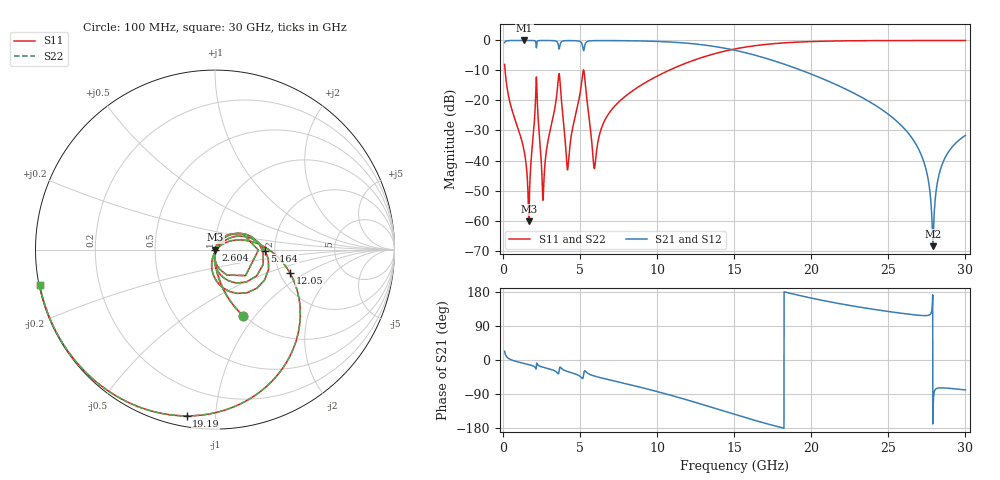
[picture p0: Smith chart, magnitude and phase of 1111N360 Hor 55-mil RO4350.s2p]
# GHz S MA R 50
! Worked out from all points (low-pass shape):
!   3201 points, 100 MHz to 30 GHz, reference 50 ohm
!   highest |S21| = -0.01 dB at 1.371 GHz (marker M1); lowest = -68.5 dB at 27.89 GHz (marker M2)
!   |S21| within 3 dB of the highest: start of sweep to 5.199 GHz; 5.253 GHz to 14.8 GHz (9.544 GHz wide, 95.2 % of centre)
!   lowest |S11| = -60.2 dB at 1.67 GHz (marker M3), VSWR 1.00, Z = 50.1 - j0.0177 ohm
!   |S11| at or under -10 dB: 130.5 MHz to 5.2 GHz (5.069 GHz wide, 190 % of centre); 5.24 GHz to 10.75 GHz (5.509 GHz wide, 68.9 % of centre)
!   |S22| runs from -60.2 to 0.0 dB; largest |S21 - S12| = 0
!   S11 on the Smith chart (normalised r, x): 100 MHz: 0.99, -0.87; 2.604 GHz: 1.00, +0.00; 5.164 GHz: 1.77, -0.02; 12.05 GHz: 2.27, -0.72; 19.19 GHz: 0.05, -0.84; 30 GHz: 0.00, -0.10
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0.1  0.3992 -67.2  0.9166 22.8  0.9166 22.8  0.3992 -67.2
1.37075  0.01424 -96.5  0.999 -9.3  0.999 -9.3  0.01424 -96.5
1.66975  0.0009785 -10.4  0.9988 -12.3  0.9988 -12.3  0.0009785 -10.4
2.146281  0.2123 16.9  0.829 -23.7  0.829 -23.7  0.2123 16.9
2.604125  0.002351 6.1  0.9976 -19.1  0.9976 -19.1  0.002351 6.1
3.585219  0.2307 14.7  0.8384 -36.4  0.8384 -36.4  0.2307 14.7
4.201906  0.007348 -6.2  0.9928 -30.6  0.9928 -30.6  0.007348 -6.2
5.089563  0.1939 21.1  0.9105 -46.9  0.9105 -46.9  0.1939 21.1
5.164313  0.2791 -1.1  0.7908 -49.1  0.7908 -49.1  0.2791 -1.1
5.939844  0.007524 -21.9  0.9923 -42.5  0.9923 -42.5  0.007524 -21.9
6.986344  0.06712 33.9  0.9936 -53.2  0.9936 -53.2  0.06712 33.9
10.06978  0.2602 5.2  0.9612 -84.1  0.9612 -84.1  0.2602 5.2
12.05066  0.4361 -17.2  0.8946 -106.7  0.8946 -106.7  0.4361 -17.2
15.05  0.7214 -54.3  0.6854 -143.9  0.6854 -143.9  0.7214 -54.3
19.18928  0.9399 -99.7  0.3298 170.7  0.3298 170.7  0.9399 -99.7
20.03956  0.9584 -107.3  0.272 163.0  0.272 163.0  0.9584 -107.3
25.01978  0.9952 -142.8  0.05837 127.9  0.05837 127.9  0.9952 -142.8
27.10344  0.9969 -154.4  0.01298 117.6  0.01298 117.6  0.9969 -154.4
27.54259  0.997 -156.6  0.005525 117.5  0.005525 117.5  0.997 -156.6
27.88831  0.997 -158.4  0.0003743 -168.9  0.0003743 -168.9  0.997 -158.4
28.53303  0.9969 -161.6  0.009152 -73.6  0.009152 -73.6  0.9969 -161.6
30  0.9966 -168.5  0.02617 -79.0  0.02617 -79.0  0.9966 -168.5
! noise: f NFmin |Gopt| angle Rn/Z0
0.1  0.0006719  0.7376  1.908  0.0005121
3.417  0.03209  0.807  24.75  0.03301
6.743  0.02133  0.5313  47.12  0.00686
10.06  0.0254  0.4658  64.1  0.006065
13.39  0.03665  0.5265  79.41  0.008584
16.7  0.05766  0.6432  95.98  0.01449
20.03  0.1044  0.7815  114.8  0.02945
23.35  0.241  0.8993  134.2  0.0806
26.67  1.24  0.9793  152.3  0.7955
30  1.012  0.974  168.4  0.09235
